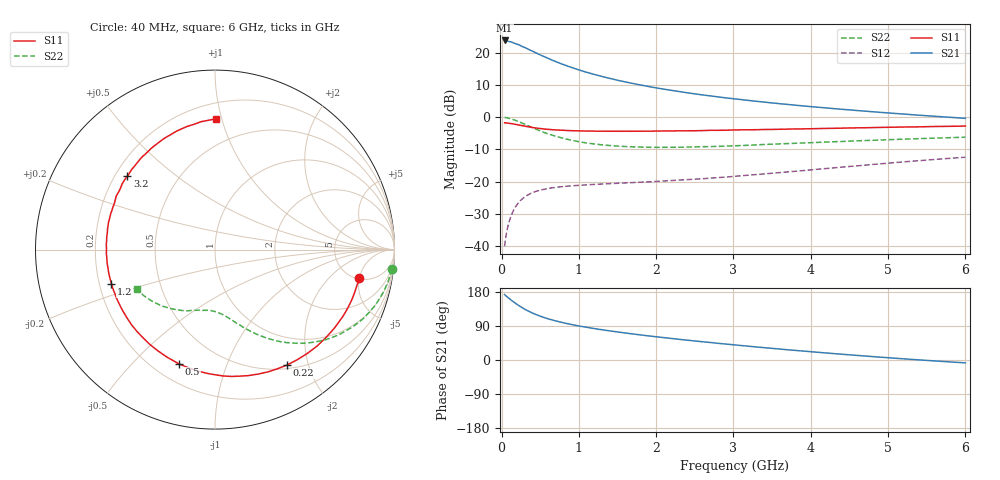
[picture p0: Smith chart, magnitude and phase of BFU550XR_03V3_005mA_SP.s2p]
! Filename:  P:\Prog\Test\Noise\ATS_data\Testdata_Net\03 Spar\BFU550XR_APG2013_45_C05_03p3V_005mA_SP_CM01_D.s2p
! Date/Time: Tue 06/Aug/2013 14:38:14
! BFU550XR_APG2013_45_C05_03p3V_1to35mA_SP_CM01_Bias4_R.s2p
! MDIF S-parameter v. bias file
! BFU550XR_APG2013_45_C05_03p3V_1to35mA_SP_CM01
! Date/time Fri Aug 02 14:41:13 2013
! VAR V_out= 3.3010
! VAR I_out= 4.9950
! VAR V_in= 0.8158
! VAR I_in= 0.0557
! Device data file deembeded for feedlines and parallel
! Original file: \03 Spar\BFU550XR_APG2013_45_C05_03p3V_005mA_SP_CM01_R.s2p
! Feed-files: PR006V01_02082013_Feed1.s2p, PR006V01_02082013_Feed2.s2p
! Parallel-file: PR006V01_02082013_Par.s2p
# MHz S MA R 50
!  Freq-MHz  S11-mag  S11-arg  S21-mag  S21-arg  S12-mag  S12-arg  S22-mag  S22-arg
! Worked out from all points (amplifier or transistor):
!   98 points, 40 MHz to 6 GHz, reference 50 ohm
!   highest |S21| = 23.8 dB at 40 MHz (marker M1)
!   |S21| within 3 dB of that: start of sweep to 370.8 MHz
!   unconditionally stable (mu >= 1): 2.374 GHz to 4.387 GHz
!   at 300 MHz: K = 0.17, MSG = 23.2 dB, |S12| = -24.7 dB
!   at 1.6 GHz: K = 0.78, MSG = 15.7 dB, |S12| = -20.4 dB
!   at 6 GHz: K = 0.86, MSG = 6.0 dB, |S12| = -12.4 dB
!   S11 on the Smith chart (normalised r, x): 40 MHz: 5.12, -4.97; 220 MHz: 0.55, -1.67; 500 MHz: 0.30, -0.69; 1.2 GHz: 0.25, -0.15; 3.2 GHz: 0.25, +0.34; 6 GHz: 0.31, +0.96
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40  0.8189 -11.3  15.46 172.8  0.01001 84.1  0.9895 -6.3
50  0.816 -14.1  15.44 170.3  0.01246 82.8  0.9864 -8.0
120  0.7962 -33.3  14.73 158.8  0.0287 72.5  0.946 -19.1
180  0.7741 -48.4  13.83 149.7  0.04059 65.0  0.8932 -27.4
220  0.7582 -58.0  13.3 144.1  0.04723 60.7  0.8544 -32.3
260  0.7424 -66.6  12.62 139.0  0.05304 56.7  0.8157 -36.9
320  0.7181 -79.1  11.75 131.9  0.06018 51.6  0.7571 -42.9
420  0.6863 -96.1  10.27 122.2  0.06896 45.1  0.6708 -50.8
500  0.6678 -107.5  9.247 115.8  0.07398 41.0  0.6137 -56.0
600  0.6475 -119.6  8.184 108.9  0.07826 37.3  0.5527 -61.3
700  0.6338 -129.4  7.28 103.2  0.08157 34.6  0.5067 -65.5
850  0.6214 -141.5  6.221 96.0  0.08529 31.9  0.4544 -70.6
1050  0.6118 -154.0  5.184 88.1  0.08847 30.0  0.4071 -76.0
1200  0.6078 -161.7  4.599 83.0  0.09071 29.3  0.3844 -79.4
1550  0.6046 -176.2  3.628 72.7  0.09506 29.1  0.3533 -86.3
2050  0.61 168.1  2.781 60.2  0.1016 31.0  0.3407 -94.9
2500  0.6161 156.2  2.298 50.2  0.1094 33.1  0.3463 -102.0
3100  0.6361 142.3  1.874 38.2  0.1236 36.3  0.3633 -110.9
3200  0.6371 140.1  1.815 36.3  0.1264 36.7  0.3671 -112.3
4100  0.6663 122.4  1.424 20.2  0.1563 37.9  0.4068 -125.7
5200  0.7037 102.7  1.118 3.1  0.203 34.7  0.456 -141.6
6000  0.7283 89.8  0.9602 -7.6  0.2393 29.9  0.4896 -153.1
